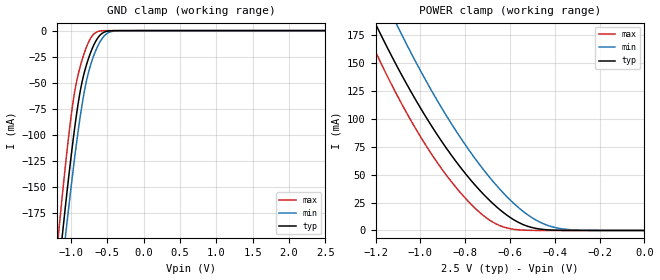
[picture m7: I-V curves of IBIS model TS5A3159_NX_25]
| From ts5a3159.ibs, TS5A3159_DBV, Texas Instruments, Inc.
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[Model]   TS5A3159_NX_25
Model_type  Terminator
| variable   typ   min   max
C_comp   24.73pF   22.58pF   25.61pF
| C_tri-state   24.73pF   22.58pF   25.61pF
[Temperature Range]   40   100   -40
| Ambient temperature   25   85   -40
[Voltage range]   2.5   2.3   2.7
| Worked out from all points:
|   GND clamp passes 1 mA (typ) near -0.53 V on its own axis
|   POWER clamp passes 1 mA (typ) near -0.46 V on its own axis
[GND Clamp]
| TS5A3159_NX_25
|   Voltage   I(typ)   I(min)   I(max)
-2.5V     -1.37A     -1.346A    -1.423A
-1.185V   -240.8mA   -268.6mA   -204.3mA
-1.165V   -227mA     -255.1mA   -189.8mA
-1.125V   -199.8mA   -228.6mA   -161.6mA
-1.07V    -164mA     -193.3mA   -124.7mA
-980mV    -109.7mA   -138.9mA   -72.24mA
-920mV    -78.26mA   -105.7mA   -47.6mA
-790mV    -33.35mA   -49.04mA   -16.11mA
-655mV    -9.563mA   -18.35mA   -1.638mA
-535mV    -1.211mA   -4.51mA    -47.67uA
-400mV    -38.46uA   -339.9uA   -258nA
2.5V      754pA      33.77uA    54.87pA
[POWER Clamp]
| TS5A3159_NX_25
|   Voltage   I(typ)   I(min)   I(max)
-2.5V     969.2mA    1.035A     1.005A
-1.25V    206mA      247.2mA    181.9mA
-1.18V    176.7mA    215.9mA    151.5mA
-1.105V   147.3mA    184.2mA    121.5mA
-1.085V   139.8mA    176.1mA    114mA
-945mV    91.98mA    123.4mA    66.81mA
-790mV    48.71mA    73.98mA    26.9mA
-675mV    23.88mA    43.76mA    7.285mA
-545mV    5.59mA     17.68mA    357.8uA
-475mV    1.513mA    8.318mA    37.05uA
-385mV    174uA      2.024mA    1.242uA
0V        0A         0A         0A
